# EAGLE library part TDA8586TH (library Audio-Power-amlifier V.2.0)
Power amplifier with load detection and auto BTL/SE selection
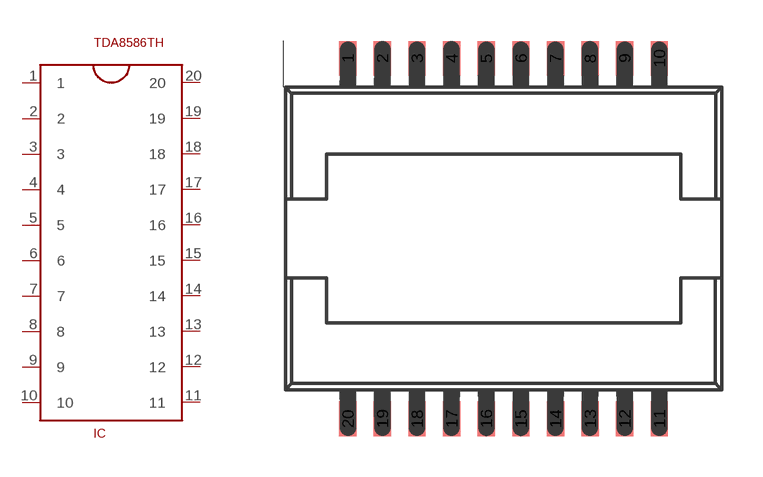
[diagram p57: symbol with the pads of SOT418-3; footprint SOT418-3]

Designator prefix IC

## TDA8586TH  [SOT418-3]
1  1  nc
2  2  in
3  3  in
4  4  in
5  5  in
6  6
7  7
8  8
9  9
10  10
11  11  out
12  12
13  13  pwr
14  14  out
15  15  pwr
16  16  pwr
17  17  out
18  18  pwr
19  19
20  20  out

## Footprint SOT418-3 (pad centres in mm)
smd 0.635 x 1.27: 1 -5.715,6.615; 2 -4.445,6.615; 3 -3.175,6.615; 4 -1.905,6.615; 5 -0.635,6.615; 6 0.635,6.615; 7 1.905,6.615; 8 3.175,6.615; 9 4.445,6.615; 10 5.715,6.615; 11 5.715,-6.615; 12 4.445,-6.615; 13 3.175,-6.615; 14 1.905,-6.615; 15 0.635,-6.615; 16 -0.635,-6.615; 17 -1.905,-6.615; 18 -3.175,-6.615; 19 -4.445,-6.615; 20 -5.715,-6.615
